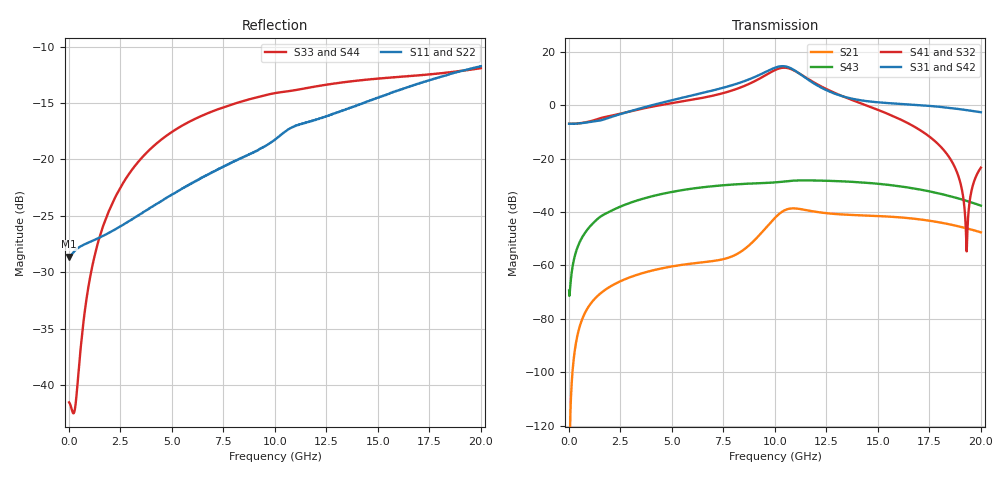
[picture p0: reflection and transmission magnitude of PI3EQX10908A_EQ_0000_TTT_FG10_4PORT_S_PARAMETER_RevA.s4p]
! NPort=4 DATA=2000 NOISE=0 GROUPDELAY=0 COMPLEX_DATAFORMAT=POLAR
! NumOfBlock=1 NumOfParam=0
! .MODEL Smodel S TSTONEFILE=PI3EQX10908A_EQ_0000_TTT_FG10_4PORT_S_PARAMETER_RevA.s4p TYPE=S
!  -- The above .MODEL line can be used for the S element in the netlist.
! The s parameter is extracted from the linear redriver, it is not bi-directional; only s(4,1)s(4,2) and s(3,1)s(3,2)
! should be the insertion loss
!Port definition:
!Port1 = input+
!Port2 = input-
!Port3 = output+
!Port4 = output-
# Hz S MA R  50
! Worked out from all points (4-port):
!   2000 points, 10 MHz to 20 GHz, reference 50 ohm
!   strongest paths, dB at 10 MHz, 5.01 GHz, 10.01 GHz, 15.01 GHz, 20 GHz:
!     S31: -6.9, 1.9, 14.1, 1.1, -2.6
!     S42: -6.9, 1.9, 14.1, 1.1, -2.6
!     S41: -6.9, 0.8, 13.2, -1.8, -23.4
!     S32: -6.9, 0.8, 13.2, -1.8, -23.4
!     S43: -69.4, -32.4, -28.9, -29.4, -37.6
!     S21: -127.3, -60.4, -42.1, -41.5, -47.6
!   lowest |S11| = -28.6 dB at 10 MHz (marker M1), VSWR 1.08, Z = 46.4 - j0.024 ohm
!   |S11| at or under -10 dB: start of sweep to end of sweep
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1e7  0.03701 -179.6  4.327e-07 13.5  0 0.0  0 0.0
     4.327e-07 13.5  0.03701 -179.6  0 0.0  0 0.0
     0.4502 -0.1  0.4502 179.9  0.008374 26.0  0.00034 -27.1
     0.4502 179.9  0.4502 -0.1  0.00034 -27.1  0.008374 26.0
8.23e9  0.1002 -116.7  0.001696 123.0  1.436e-06 47.9  5.038e-07 132.2
        0.001696 123.0  0.1002 -116.7  5.038e-07 132.2  1.436e-06 47.9
        2.586 -53.5  2.078 119.8  0.179 0.0  0.03325 0.5
        2.078 119.8  2.586 -53.5  0.03325 0.5  0.179 0.0
1.002e10  0.1229 -110.5  0.007909 120.8  5.727e-06 1.6  3.61e-06 123.9
          0.007909 120.8  0.1229 -110.5  3.61e-06 123.9  5.727e-06 1.6
          5.067 -107.9  4.582 66.6  0.1969 -13.0  0.03595 -16.1
          4.582 66.6  5.067 -107.9  0.03595 -16.1  0.1969 -13.0
1.075e10  0.1377 -111.0  0.01163 82.2  6.776e-06 -32.5  7.265e-06 84.5
          0.01163 82.2  0.1377 -111.0  7.265e-06 84.5  6.776e-06 -32.5
          4.974 -153.8  4.802 18.2  0.2013 -17.6  0.03836 -23.9
          4.802 18.2  4.974 -153.8  0.03836 -23.9  0.2013 -17.6
1.187e10  0.149 -112.2  0.01028 42.4  6.147e-06 -38.6  1.035e-05 38.6
          0.01028 42.4  0.1491 -112.2  1.035e-05 38.6  6.147e-06 -38.6
          2.597 165.3  2.706 -31.1  0.2096 -23.4  0.03902 -38.9
          2.706 -31.1  2.597 165.3  0.03902 -38.9  0.2096 -23.4
1.485e10  0.1855 -110.5  0.008476 0.4  2.385e-05 -56.4  2.547e-05 -27.4
          0.008476 0.4  0.1856 -110.5  2.547e-05 -27.4  2.385e-05 -56.4
          1.149 141.2  0.8634 -90.3  0.2277 -38.0  0.03428 -75.6
          0.8634 -90.3  1.149 141.2  0.03428 -75.6  0.2277 -38.0
2e10  0.2591 -113.6  0.004169 -57.5  9.279e-05 -148.1  7.178e-05 -136.3
      0.004169 -57.5  0.2592 -113.6  7.178e-05 -136.3  9.278e-05 -148.1
      0.7392 66.2  0.06791 -10.9  0.254 -52.2  0.01319 -136.9
      0.06792 -10.9  0.7391 66.2  0.01319 -136.9  0.254 -52.2
